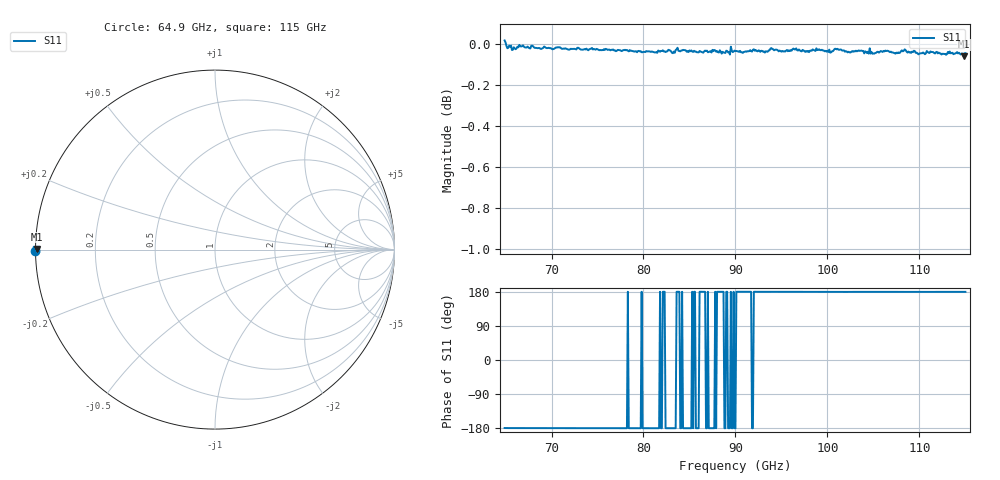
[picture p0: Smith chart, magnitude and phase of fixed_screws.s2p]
# GHz S MA R 50
!freq magS11 angS11
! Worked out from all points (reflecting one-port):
!   502 points, 64.9 GHz to 115 GHz, reference 50 ohm
!   lowest |S11| = -0.1 dB at 114.8 GHz (marker M1), VSWR 284.64, Z = 0.176 + j0.0839 ohm
!   phase of S11 starts at -179 deg and turns -1 deg over the sweep
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64.9  1.002 -179.5
65.4  0.9989 -179.6
65.9  0.9979 -179.6
66.7  0.9984 -179.6
71.2  0.9971 -179.8
77.5  0.9962 -179.9
83.3  0.9955 -179.9
83.7  0.9977 179.9
84.9  0.9953 -179.9
86.5  0.9949 180.0
87.4  0.995 -179.9
88.5  0.9944 180.0
89.2  0.9951 -179.9
90  0.9958 -180.0
92  0.9968 180.0
93.2  0.995 179.9
94  0.997 180.0
95.2  0.9956 179.9
96.3  0.9972 180.0
100.3  0.9949 179.9
101  0.9968 179.8
102.5  0.995 179.7
103.2  0.9957 179.9
108.8  0.9955 179.7
110.1  0.9945 179.8
113.9  0.9945 179.7
114.8  0.993 179.8
115  0.9946 179.8
